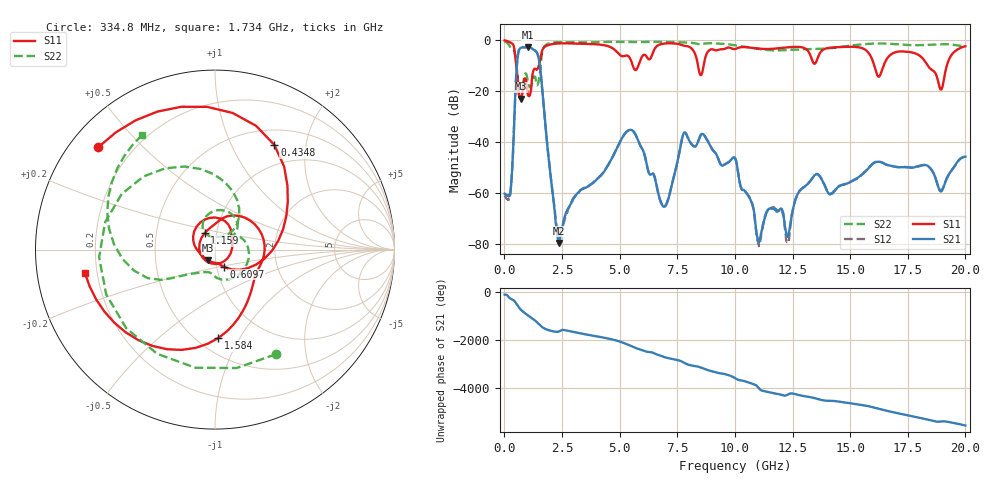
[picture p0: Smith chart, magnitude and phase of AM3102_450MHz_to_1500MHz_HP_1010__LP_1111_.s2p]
!Agilent Technologies,E8364B,MY43040894,A.07.50.67
!Agilent E8364B: A.07.50.67
!Date: Thursday, January 11, 2018 06:21:53
!Correction: S11(Full 2 Port(1,2))
!S21(Full 2 Port(1,2))
!S12(Full 2 Port(1,2))
!S22(Full 2 Port(1,2))
!S2P File: Measurements: S11, S21, S12, S22:
# Hz S  dB  R 50
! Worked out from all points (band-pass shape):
!   1601 points, 10 MHz to 20 GHz, reference 50 ohm
!   highest |S21| = -2.74 dB at 1.022 GHz (marker M1); lowest = -79.7 dB at 2.359 GHz (marker M2)
!   |S21| within 3 dB of the highest: 587.7 MHz to 1.452 GHz (864.6 MHz wide, 84.8 % of centre)
!   lowest |S11| = -23.0 dB at 709.6 MHz (marker M3), VSWR 1.15, Z = 45.9 - j5.43 ohm
!   |S11| at or under -10 dB: 522.5 MHz to 1.491 GHz (968 MHz wide, 96.2 % of centre); 16.05 GHz to 16.45 GHz (399.7 MHz wide, 2.46 % of centre); 18.37 GHz to 19.19 GHz (818.9 MHz wide, 4.36 % of centre)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
!   |S22| runs from -23.0 to -0.5 dB; largest |S21 - S12| = 0.0018
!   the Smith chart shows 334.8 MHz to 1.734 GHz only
!   S11 on the Smith chart (normalised r, x): 334.8 MHz: 0.08, +0.37; 434.8 MHz: 0.70, +1.48; 609.7 MHz: 1.08, -0.21; 1.159 GHz: 0.88, +0.16; 1.584 GHz: 0.63, -0.82; 1.734 GHz: 0.15, -0.09
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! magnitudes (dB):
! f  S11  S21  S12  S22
! 10 MHz  -0.1  -60.2  -61.2  -0.5
! 334.8 MHz  -1.3  -51.2  -51.0  -3.4
! 434.8 MHz  -3.5  -29.8  -29.6  -4.4
! 609.7 MHz  -19.5  -4.5  -4.5  -19.0
! 709.6 MHz  -23.0  -3.0  -3.0  -23.0
! 1.022 GHz  -21.4  -2.7  -2.7  -16.3
! 1.159 GHz  -19.3  -3.0  -3.0  -18.1
! 1.584 GHz  -6.1  -13.6  -13.6  -9.3
! 1.734 GHz  -2.7  -28.9  -28.9  -2.4
! 2.359 GHz  -1.2  -79.7  -76.3  -0.7
! 3.346 GHz  -1.4  -58.7  -58.6  -0.8
! 5.47 GHz  -7.4  -35.2  -35.2  -0.7
! 6.682 GHz  -1.9  -60.3  -60.6  -0.6
! 7.819 GHz  -2.2  -36.3  -36.2  -0.8
! 10.01 GHz  -3.4  -46.4  -46.3  -1.9
! 11.03 GHz  -3.3  -79.2  -79.7  -3.4
! 11.63 GHz  -3.3  -66.2  -65.7  -3.9
! 12.3 GHz  -2.7  -77.3  -79.6  -3.8
! 13.34 GHz  -7.5  -54.5  -54.5  -3.4
! 16.68 GHz  -6.3  -49.2  -49.1  -1.3
! 18.94 GHz  -19.4  -59.4  -59.1  -1.5
! 20 GHz  -2.3  -45.7  -45.7  -2.4
